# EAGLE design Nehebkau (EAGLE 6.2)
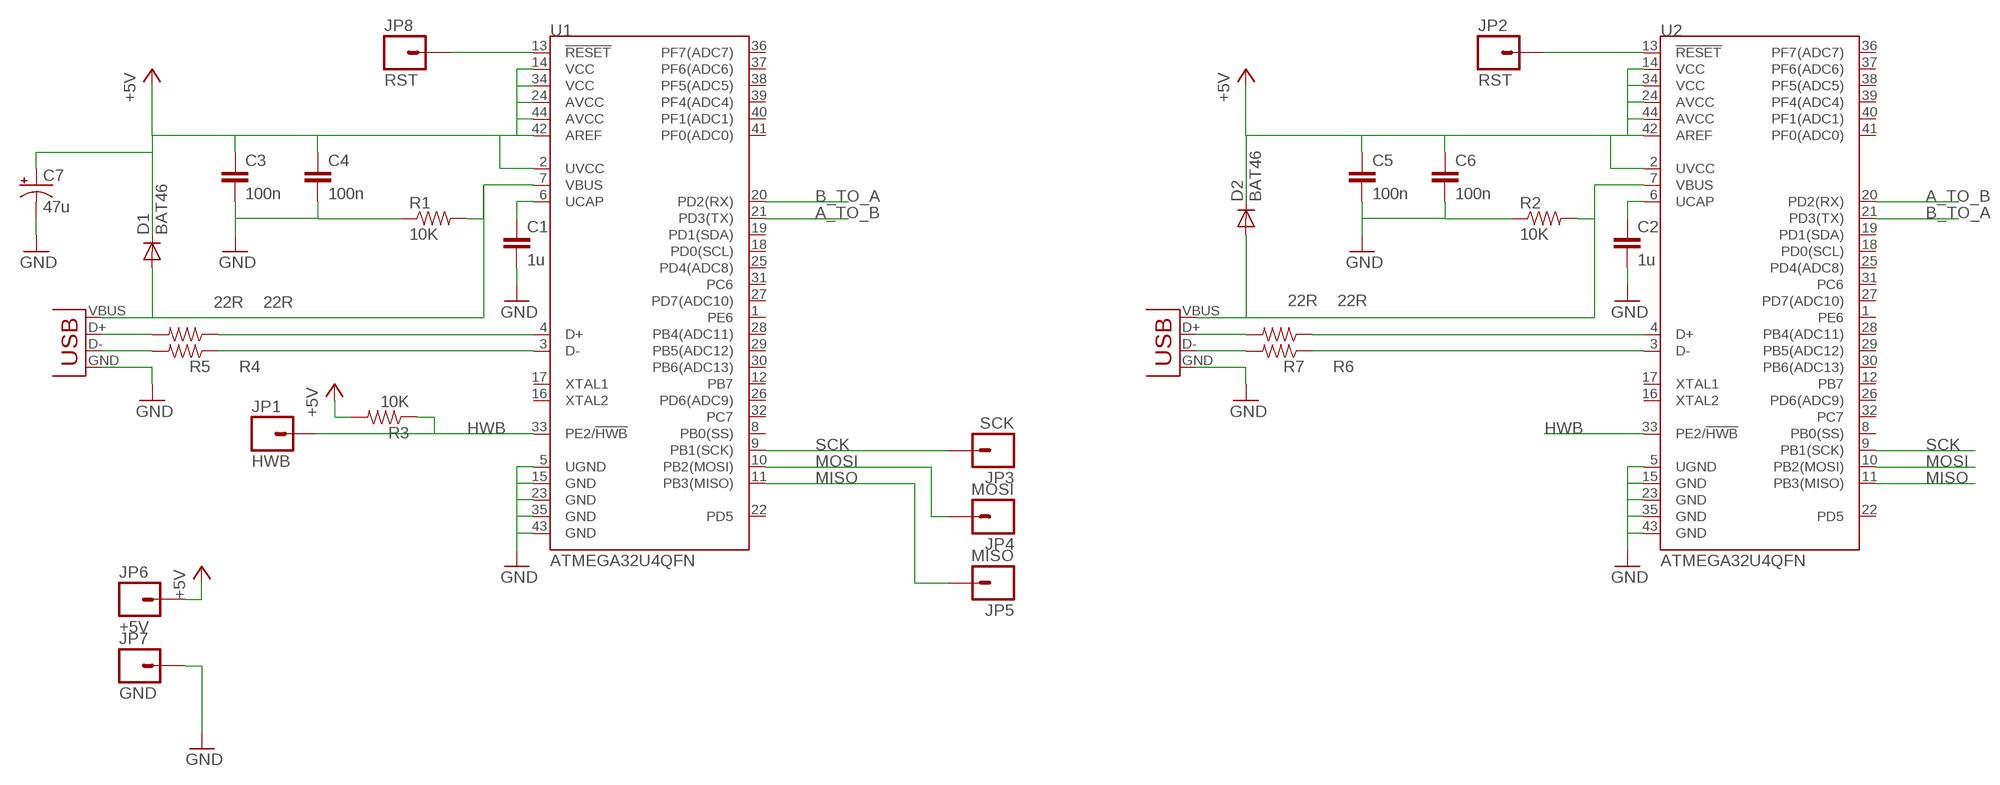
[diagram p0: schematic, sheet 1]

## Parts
C1  1u  CAP0603-CAP  [0603-CAP]
C2  1u  CAP0603-CAP  [0603-CAP]
C3  100n  CAP0603-CAP  [0603-CAP]
C4  100n  CAP0603-CAP  [0603-CAP]
C5  100n  CAP0603-CAP  [0603-CAP]
C6  100n  CAP0603-CAP  [0603-CAP]
C7  47u  CAP_POL3528-KIT  [EIA3528-KIT]
D1  BAT46  DIODEMINIMELF  [MINIMELF]
D2  BAT46  DIODEMINIMELF  [MINIMELF]
JP1  HWB  M01PTH  [1X01]
JP2  RST  M01PTH  [1X01]
JP3  SCK  M01PTH  [1X01]
JP4  MOSI  M01PTH  [1X01]
JP5  MISO  M01PTH  [1X01]
JP6  +5V  M01PTH  [1X01]
JP7  GND  M01PTH  [1X01]
JP8  RST  M01PTH  [1X01]
R1  10K  RESISTOR0603-RES  [0603-RES]
R2  10K  RESISTOR0603-RES  [0603-RES]
R3  10K  RESISTOR0603-RES  [0603-RES]
R4  22R  RESISTOR0603-RES  [0603-RES]
R5  22R  RESISTOR0603-RES  [0603-RES]
R6  22R  RESISTOR0603-RES  [0603-RES]
R7  22R  RESISTOR0603-RES  [0603-RES]
U1  ATMEGA32U4QFN  [QFN-44]
U2  ATMEGA32U4QFN  [QFN-44]
X1  USB-A-H  [USB-A-H]
X2  USB-A-H  [USB-A-H]

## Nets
+5V: C3.1 C4.1 C5.1 C6.1 C7.A(+) D1.C D2.C JP6.1 R3.2 U1.2(UVCC) U1.14(VCC) U1.24(AVCC) U1.34(VCC) U1.42(AREF) U1.44(AVCC) U2.2(UVCC) U2.14(VCC) U2.24(AVCC) U2.34(VCC) U2.42(AREF) U2.44(AVCC)
A_TO_B: U1.21(PD3(TX)) U2.20(PD2(RX))
B_TO_A: U1.20(PD2(RX)) U2.21(PD3(TX))
GND: C1.2 C2.2 C3.2 C4.2 C5.2 C6.2 C7.C(-) JP7.1 R1.1 R2.1 U1.5(UGND) U1.15(GND) U1.23(GND) U1.35(GND) U1.43(GND) U2.5(UGND) U2.15(GND) U2.23(GND) U2.35(GND) U2.43(GND) X1.GND(VBUS) X2.GND(VBUS)
HWB: JP1.1 R3.1 U1.33(PE2/!HWB) U2.33(PE2/!HWB)
MISO: JP5.1 U1.11(PB3(MISO)) U2.11(PB3(MISO))
MOSI: JP4.1 U1.10(PB2(MOSI)) U2.10(PB2(MOSI))
N$1: C2.1 U2.6(UCAP)
N$2: C1.1 U1.6(UCAP)
N$3: R6.2 X2.D+(D-)
N$4: R7.2 X2.D-(D+)
N$5: R4.2 X1.D+(D-)
N$6: R5.2 X1.D-(D+)
N$7: R4.1 U1.4(D+)
N$8: R5.1 U1.3(D-)
N$9: R6.1 U2.4(D+)
N$10: R7.1 U2.3(D-)
N$11: JP8.1 U1.13(!RESET)
RST: JP2.1 U2.13(!RESET)
SCK: JP3.1 U1.9(PB1(SCK)) U2.9(PB1(SCK))
VBUS_A: D1.A R1.2 U1.7(VBUS) X1.VBUS(GND)
VBUS_B: D2.A R2.2 U2.7(VBUS) X2.VBUS(GND)
Unconnected: U1.1(PE6) U1.8(PB0(SS)) U1.12(PB7) U1.16(XTAL2) U1.17(XTAL1) U1.18(PD0(SCL)) U1.19(PD1(SDA)) U1.22(PD5) U1.25(PD4(ADC8)) U1.26(PD6(ADC9)) U1.27(PD7(ADC10)) U1.28(PB4(ADC11)) U1.29(PB5(ADC12)) U1.30(PB6(ADC13)) U1.31(PC6) U1.32(PC7) U1.36(PF7(ADC7)) U1.37(PF6(ADC6)) U1.38(PF5(ADC5)) U1.39(PF4(ADC4)) U1.40(PF1(ADC1)) U1.41(PF0(ADC0)) U2.1(PE6) U2.8(PB0(SS)) U2.12(PB7) U2.16(XTAL2) U2.17(XTAL1) U2.18(PD0(SCL)) U2.19(PD1(SDA)) U2.22(PD5) U2.25(PD4(ADC8)) U2.26(PD6(ADC9)) U2.27(PD7(ADC10)) U2.28(PB4(ADC11)) U2.29(PB5(ADC12)) U2.30(PB6(ADC13)) U2.31(PC6) U2.32(PC7) U2.36(PF7(ADC7)) U2.37(PF6(ADC6)) U2.38(PF5(ADC5)) U2.39(PF4(ADC4)) U2.40(PF1(ADC1)) U2.41(PF0(ADC0))

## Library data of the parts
C1-C6 = Nehebkau:CAP: Capacitor
C7 = Nehebkau:CAP_POL: Capacitor Polarized
D1 D2 = Nehebkau:DIODE: Diode
JP1-JP8 = Nehebkau:M01: Header 1
R1-R7 = Nehebkau:RESISTOR: Resistor
U1 U2 = Nehebkau:ATMEGA32U4
X1 X2 = Nehebkau:USB: USB Connectors USB-B-PTH is fully proven SKU : PRT-00139 USB-miniB is fully proven SKU : PRT-00587 USB-A-PCB is untested. USB-A-H is throughly reviewed, but untested. Spark Fun Electronics SKU : PRT-00437 USB-B-SMT is throughly reviewed, but untested. Needs silkscreen touching up. USB-A-S has not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

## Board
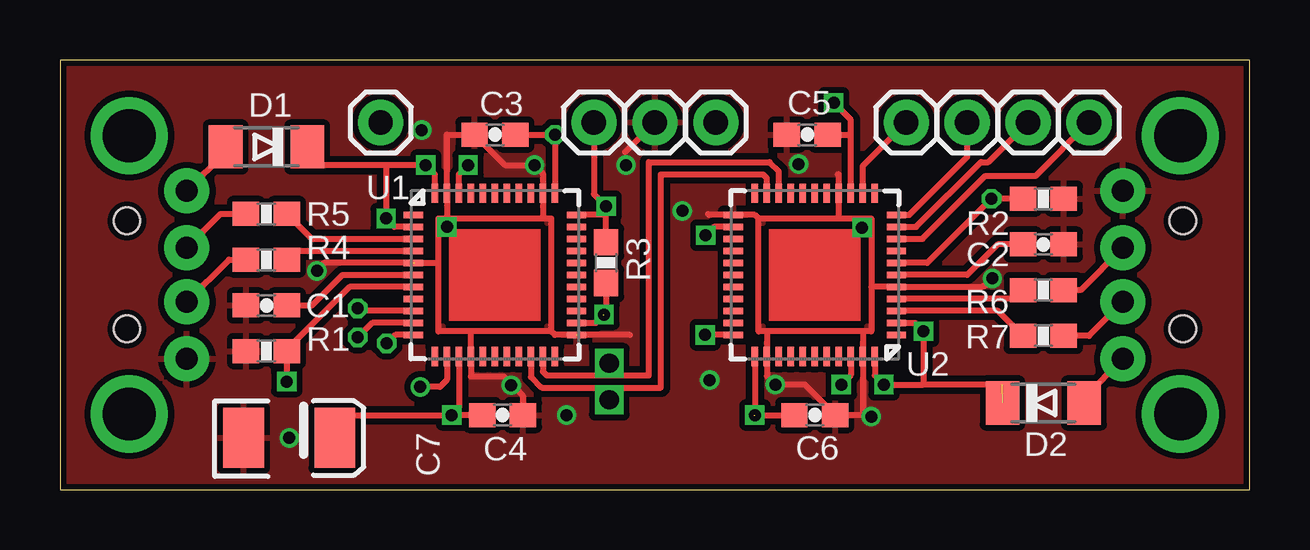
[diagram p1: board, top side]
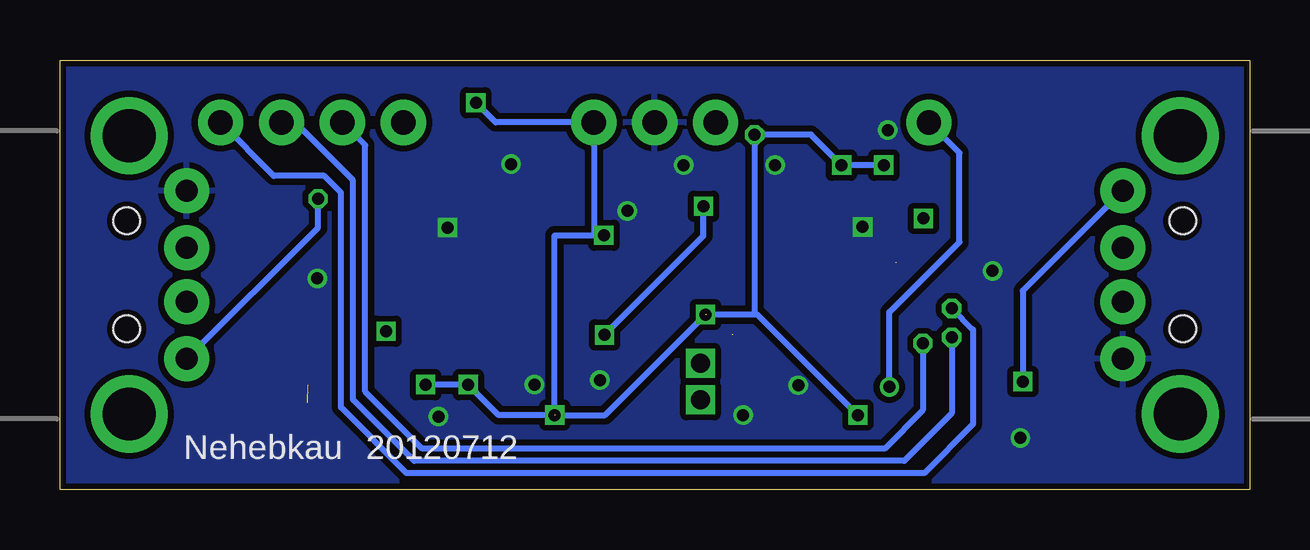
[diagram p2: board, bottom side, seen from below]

Size 49.59 x 17.91 mm. Coordinates in mm from the lower left corner, seen from the top.
Outline: 0,0 49.59,0 49.59,17.91 0,17.91 0,0
Copper layers (1*16): Top 0.035mm / dielectric 1.5mm / Bottom 0.035mm
Design rules: minimum track width 6mil, minimum drill 0.3mm, track to track 7mil, track to pad 7mil, pad to pad 7mil, via to via 7mil, smd to smd 0mil, copper to edge 10mil, drill to drill 10mil, minimum pad ring 10mil, minimum via ring 6mil, stop-mask expansion 2mil, vias tented up to drill 25mil, thermal gap 10mil

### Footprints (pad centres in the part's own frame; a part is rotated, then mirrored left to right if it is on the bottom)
0603-CAP = smd 1.1 x 1: 1 -0.85,0; 2 0.85,0
EIA3528-KIT = smd 1.7 x 2.5: A 1.9,0; C -1.9,0
MINIMELF = smd 1.4 x 1.8: A 1.7,0; C -1.7,0
1X01 = drill 1.016 pad 1.88: 1 0,0
0603-RES = smd 1.1 x 1: 1 -0.85,0; 2 0.85,0
QFN-44 = smd 0.8 x 0.279: 1 -3.4,2.5; 2 -3.4,2; 3 -3.4,1.5; 4 -3.4,1; 5 -3.4,0.5; 6 -3.4,0; 7 -3.4,-0.5; 8 -3.4,-1; 9 -3.4,-1.5; 10 -3.4,-2; 11 -3.4,-2.5; 23 3.4,-2.5; 24 3.4,-2; 25 3.4,-1.5; 26 3.4,-1; 27 3.4,-0.5; 28 3.4,0; 29 3.4,0.5; 30 3.4,1; 31 3.4,1.5; 32 3.4,2; 33 3.4,2.5 | smd 0.279 x 0.8: 12 -2.5,-3.4; 13 -2,-3.4; 14 -1.5,-3.4; 15 -1,-3.4; 16 -0.5,-3.4; 17 0,-3.4; 18 0.5,-3.4; 19 1,-3.4; 20 1.5,-3.4; 21 2,-3.4; 22 2.5,-3.4; 34 2.5,3.4; 35 2,3.4; 36 1.5,3.4; 37 1,3.4; 38 0.5,3.4; 39 0,3.4; 40 -0.5,3.4; 41 -1,3.4; 42 -1.5,3.4; 43 -2,3.4; 44 -2.5,3.4
USB-A-H = drill 0.914 pad 1.88: D+ 2.4,1.127; D- 2.4,-1.127; GND 2.4,3.5; VBUS 2.4,-3.5 | drill 2.2: GND2 0,-5.8; GND3 0,5.8 | hole 1.1: -0.1,2.25; -0.1,-2.25

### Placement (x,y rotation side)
C1  8.6,7.68 180 top
C2  40.99,10.22 0 top
C3  18.13,14.8 180 top
C4  18.45,3.11 0 top
C5  31.15,14.8 180 top
C6  31.46,3.11 0 top
C7  9.56,2.16 0 top
D1  8.6,14.29 180 top
D2  40.99,3.62 0 top
JP1  22.26,15.3 0 top
JP2  35.27,15.3 0 top
JP3  42.89,15.3 0 top
JP4  40.35,15.3 0 top
JP5  37.81,15.3 0 top
JP6  27.34,15.3 0 top
JP7  24.8,15.3 0 top
JP8  13.37,15.3 0 top
R1  8.6,5.78 0 top
R2  40.99,12.13 180 top
R3  22.76,9.46 270 top
R4  8.6,9.59 180 top
R5  8.6,11.49 180 top
R6  40.99,8.32 0 top
R7  40.99,6.41 0 top
U1  18.13,8.95 0 top
U2  31.46,8.95 180 top
X1  2.89,8.95 180 bottom
X2  46.7,8.95 0 bottom

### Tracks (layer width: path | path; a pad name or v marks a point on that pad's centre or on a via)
+5V  (via drill 0.5)  (3 unrouted)
  Top 0.254: C3.1 v20.63,14.8 U1.34 | U1.24 22.33,6.95 v22.68,7.3 22.77,7.39 R3.2 | U1.42 16.63,13.14 v17.01,13.53 | U1.44 15.63,13.14 v15.25,13.53 13.6,13.53 | U1.2 13.95,10.95 v13.6,11.3 13.6,13.53 | U2.44 33.96,4.76 v34.35,4.38 36,4.38 | U2.42 32.96,4.78 v32.57,4.38 | U2.2 35.65,6.95 v36,6.6 36,4.38 | U2.24 27.27,10.95 v26.92,10.6 | U2.34 v28.96,3.11 C6.1 | U1.14 16.63,3.41 v16.33,3.11 | C4.1 v16.33,3.11 | U2.14 32.96,14.8 | C7.A 11.77,3.11 v16.33,3.11 | 39.26,4.38 36,4.38 | 13.6,13.53 10.3,13.53 D1.C | v32.25,16.13 32.96,15.41 32.96,15.24 32.96,14.8 | C5.1 32.96,14.8
  Bottom 0.254: v15.25,13.53 v17.01,13.53 18.28,14.8 v20.63,14.8 20.63,7.3 v22.68,7.3 26.87,3.11 v28.96,3.11 | v28.96,3.11 31.3,3.11 v32.57,4.38 v34.35,4.38 | v28.96,3.11 28.96,10.6 v26.92,10.6 27.34,10.6 JP6.1 31.43,15.3 v32.25,16.13 | 28.92,3.11 28.86,3.11 | v16.33,3.11 20.52,7.3 22.64,7.3
A_TO_B
  Top 0.254: U1.21 20.13,4.92 20.29,4.76 24.54,4.76 24.54,13.65 29.58,13.65 29.96,13.27 U2.20
B_TO_A
  Top 0.254: U2.21 29.46,12.99 29.3,13.14 25.05,13.14 25.05,4.25 20.08,4.25 19.63,4.71 U1.20
GND  (via drill 0.5)  (2 unrouted)
  Top 0.254: U1.5 11.01,9.45 10.51,8.95 | 16.1,11.3 16.13,11.3 U1.43 16.13,14.8 C3.2 18.55,13.53 v19.78,13.53 20.13,13.18 U1.35 20.13,11.34 20.1,11.3 | 17.11,6.6 17.13,6.6 U1.15 17.13,4.72 18.5,4.72 19.3,3.92 C4.2 | U1.23 20.63,6.45 20.48,6.6 | 23.75,6.45 21.58,6.45 | 29.46,6.57 U2.35 29.46,4.73 v29.81,4.38 31.04,4.38 C6.2 33.46,3.11 U2.43 33.46,6.57 | U2.5 38.39,8.45 arc90 38.64,8.7 | 32.42,13.14 32.46,13.14 U2.15 32.46,11.34 | 29.11,11.3 28.96,11.45 27.06,11.45 27.02,11.49 | JP7.1 23.56,14.06 | 20.48,6.6 20.48,11.3 15.78,11.3 15.78,6.6 20.48,6.6 | 14.76,9.45 15.78,9.45 | 29.11,11.3 29.11,6.6 33.81,6.6 33.81,11.3 29.11,11.3
  other vias: 9.56,2.16 15.08,14.99 23.59,13.53 25.94,11.62 27.08,4.57 21.11,3.11 33.81,3.05 30.79,13.57 38.86,8.81 10.71,9.12 18.81,4.35 16.13,10.95 33.43,10.92
  pour Top (isolate 0.254): 0,0 0,20.32 50.83,20.32 50.83,0
  pour Bottom (isolate 0.254): 0,0 0,20.32 50.83,20.32 50.83,0
HWB  (via drill 0.5)
  Top 0.254: R3.1 22.77,11.45 | 22.77,11.45 U1.33 | 22.77,11.45 v22.77,11.81 22.26,12.32 JP1.1 | U2.33 v26.89,6.45
  Bottom 0.254: v26.89,6.45 22.77,10.58 v22.77,11.81
MISO  (via drill 0.5)
  Top 0.254: U1.11 13.98,6.45 v13.62,6.1 | U2.11 35.4,11.45 37.81,13.87 JP5.1
  Bottom 0.254: v13.62,6.1 13.62,3.3 15.21,1.71 34.49,1.71 36.86,4.09 36.86,14.35 JP5.1
MOSI  (via drill 0.5)
  Top 0.254: U1.10 13.02,6.95 v12.41,6.35 | U2.10 35.69,10.95 38.39,13.65 38.7,13.65 JP4.1
  Bottom 0.254: v12.41,6.35 12.41,3.18 14.39,1.21 34.82,1.21 37.37,3.76 37.37,12.89 39.78,15.3 JP4.1
N$1
  Top 0.254: C2.1 39.08,10.22 37.81,8.95 U2.6
N$2
  Top 0.254: C1.1 10.51,7.68 11.78,8.95 U1.6
N$3
  Top 0.254: X2.D+ 42.54,8.32 R6.2
N$4
  Top 0.254: X2.D- 42.89,6.41 R7.2
N$5
  Top 0.254: X1.D+ 7.05,9.59 R4.2
N$6
  Top 0.254: X1.D- 6.7,11.49 R5.2
N$7
  Top 0.254: R4.1 9.82,9.95 U1.4
N$8
  Top 0.254: R5.1 10.49,10.45 U1.3
N$9
  Top 0.254: R6.1 39.77,7.95 U2.4
N$10
  Top 0.254: R7.1 39.1,7.45 U2.3
N$11  (via drill 0.5)
  Top 0.254: U1.13 16.13,4.57 15.84,4.29 v15.02,4.29
  Bottom 0.254: v15.02,4.29 15.02,7.4 12.1,10.32 12.1,14.03 JP8.1
N$12
  Top 0.254: 34.64,8.45 33.81,8.45
N$13  (via drill 0.8)
  other vias: 22.89,5.27
N$14  (via drill 0.8)
  other vias: 22.89,3.75
RST
  Top 0.254: U2.13 33.46,13.49 JP2.1
SCK  (via drill 0.5)
  Top 0.254: U1.9 12.52,7.45 v12.41,7.56 | U2.9 35.95,10.45 38.58,13.08 40.67,13.08 JP3.1
  Bottom 0.254: v12.41,7.56 11.53,6.67 11.53,2.74 13.57,0.7 35.15,0.7 37.88,3.43 37.88,12.38 38.58,13.08 40.67,13.08 JP3.1
VBUS_A  (via drill 0.5)
  Top 0.254: v9.45,4.51 R1.2 9.45,5.84 12.07,8.45 U1.7 | X1.VBUS 6.9,14.07 D1.A
  Bottom 0.254: X1.VBUS 9.45,8.29 v9.45,4.51
VBUS_B  (via drill 0.5)
  Top 0.254: R2.2 v38.83,12.13 36.16,9.45 U2.7 | X2.VBUS 42.69,3.84 D2.A
  Bottom 0.254: X2.VBUS 38.83,10.93 v38.83,12.13

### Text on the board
bNames: 20120712 | Nehebkau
